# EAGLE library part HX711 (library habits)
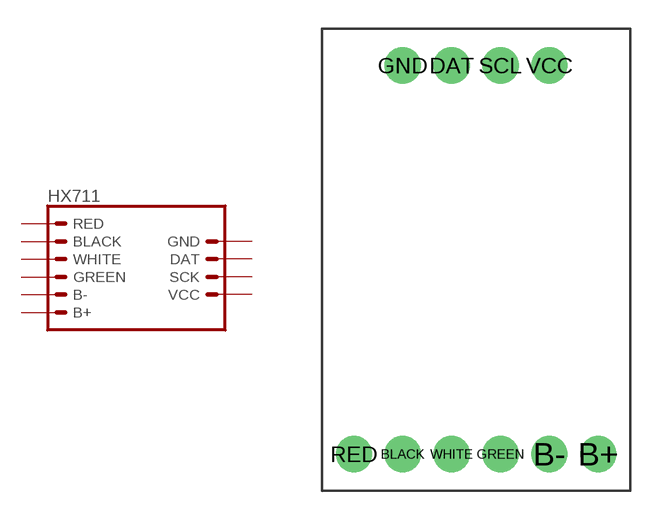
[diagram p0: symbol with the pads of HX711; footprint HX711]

Designator prefix -

## HX711  [HX711]
B+  B+  pas
B-  B-  pas
BLACK  BLACK  pas
DAT  DAT  pas
GND  GND  pas
GREEN  GREEN  pas
RED  RED  pas
SCL  SCK  pas
VCC  VCC  pwr
WHITE  WHITE  pas

## Footprint HX711 (pad centres in mm)
Plated Through Hole - 2x6 Specifications: Pin count:12 Pin pitch:0.1" Example device(s): CONN_06x2
drill 1.016 pad 1.88: B+ 6.35,-10.1; B- 3.81,-10.1; BLACK -3.81,-10.1; DAT -1.27,10.1; GND -3.81,10.1; GREEN 1.27,-10.1; RED -6.35,-10.1; SCL 1.27,10.1; VCC 3.81,10.1; WHITE -1.27,-10.1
